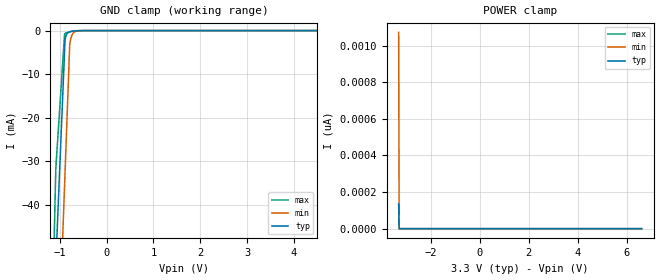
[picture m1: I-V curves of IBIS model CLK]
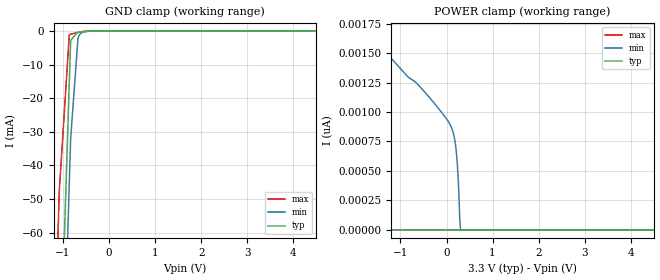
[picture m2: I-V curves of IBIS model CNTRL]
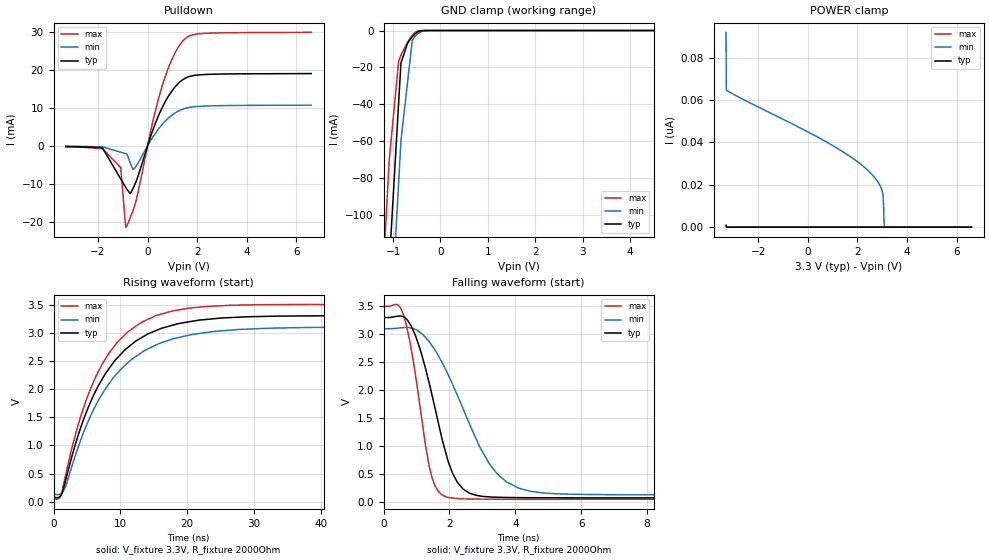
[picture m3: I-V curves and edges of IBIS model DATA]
|Texas Instruments Incorporated
| Marketing part#   Digital Voltage Range   Package-type   #pins
|   TPS544C20   3.1V -3.5V   LQFN   40
[IBIS Ver]   4.1
[File name]   tps544c20.ibs
[File Rev]   1.0
[Date]   02/18/2016
[Source]
| Texas Instruments Incorporated.
| 12500 TI Blvd
| Dallas, TX -75243
[Notes]   Revision History:
| Rev 1.0: 02/18/2016
| - Initial version of the model
| - Model generated from simulations in TISPICE
| - C_comp although listed in numerical order of value are
|   obtained from varying PVT conditions. For PVT conditions for
|   each specific value refer the buffer description under
|   respective [Model]. IBIS model user is responsible for using
|   appropriate C_comp to simulate for Signal Integrity.
| - Warnings regarding combined Non-monotonicity of various models have been
|   reviewd and considered minor and can be ignored.
[Disclaimer]
| This model is designed as an aid for customers of Texas Instruments.
| TI and its licensors and suppliers make no warranties, either expressed
| or implied, with respect to this  model, including the warranties of
| merchantability or fitness for a particular purpose. The model is
| provided solely on an "as is" basis. The entire risk as to its quality
| and performance is with the customer.
[Copyright]
 (C) Copyright 2016 Texas Instruments Incorporated.All rights reserved.
|   Device
[Component]   TPS544C20
[Manufacturer]   TI
[Package]
| variable   typ   min   max
R_pkg   0.2   0.16   0.24
L_pkg   1.5nH   1.2nH   1.8nH
C_pkg   0.4pF   0.32pF   0.48pF
[Pin]  signal_name   model_name   R_pin   L_pin   C_pin
1   CNTL   CNTRL   NA   NA   NA
2   ADDR1   NC   NA   NA   NA
3   ADDR0   NC   NA   NA   NA
4   DATA   DATA   NA   NA   NA
5   CLK   CLK   NA   NA   NA
6   SMBALERTB   SMBALERT   NA   NA   NA
7   BOOT   NC   NA   NA   NA
8   SW   NC   NA   NA   NA
9   SW   NC   NA   NA   NA
10   SW   NC   NA   NA   NA
11   SW   NC   NA   NA   NA
12   SW   NC   NA   NA   NA
13   AGNDSNS   GND   NA   NA   NA
14   GND   GND   NA   NA   NA
15   GND   GND   NA   NA   NA
16   GND   GND   NA   NA   NA
17   GND   GND   NA   NA   NA
18   GND   GND   NA   NA   NA
19   GND   GND   NA   NA   NA
20   GND   GND   NA   NA   NA
21   VIN   NC   NA   NA   NA
22   VIN   NC   NA   NA   NA
23   VIN   NC   NA   NA   NA
24   VIN   NC   NA   NA   NA
25   VIN   NC   NA   NA   NA
26   PGND   GND   NA   NA   NA
27   BP3   POWER   NA   NA   NA
28   BP6   POWER   NA   NA   NA
29   VDD   POWER   NA   NA   NA
30   BPEXT   NC   NA   NA   NA
31   VOUTS+   NC   NA   NA   NA
32   VOUTS-   NC   NA   NA   NA
33   DIFFO   NC   NA   NA   NA
34   FB   NC   NA   NA   NA
35   COMP   NC   NA   NA   NA
36   PGOOD   NC   NA   NA   NA
37   TSNS   NC   NA   NA   NA
38   AGND   GND   NA   NA   NA
39   MODE   NC   NA   NA   NA
40   RT   NC   NA   NA   NA
| Models and submodels in the file (4): CLK (Input), CNTRL (Input), DATA (I/O_open_drain), SMBALERT (Open_drain)
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|   Model
[Model]   CLK
Model_type   Input
Vinl = 0.99
Vinh = 2.31
|   typ   min   max
C_comp   0.057pF   0.055pF   0.060pF
[Voltage Range]   3.3   3.1   3.5
[Temperature Range]   25   125   -40
[Power Clamp Reference]   3.3   3.1   3.5
[GND Clamp Reference]   0   0   0
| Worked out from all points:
|   GND clamp passes 1 mA (typ) near -0.86 V on its own axis
[GND Clamp]
|   Voltage   I(typ)   I(min)   I(max)
-3.3V     -1.121A    -1.154A    -1.103A
-1.825V   -397.6mA   -433.8mA   -376.6mA
-1.082V   -53.42mA   -90.58mA   -31.68mA
-894.3mV  -4.553mA   -35.25mA   -727.9uA
-884.4mV  -1.981mA   -32.34mA   -661.1uA
-864.6mV  -1.187mA   -26.51mA   -557.5uA
-834.9mV  -611.3uA   -17.77mA   -438.9uA
-785.4mV  -279.6uA   -3.211mA   -286.8uA
-765.6mV  -218.9uA   -2.042mA   -236.7uA
-735.9mV  -154.8uA   -1.024mA   -172uA
-656.7mV  -57.61uA   -188.9uA   -58.46uA
6.6V      0A         0A         0A
[POWER Clamp]
|   Voltage   I(typ)   I(min)   I(max)
-3.3V     135.7pA    1.072nA    121.6pA
-3.28V    0A         0A         0A
-3.27V    0A         0A         0A
6.6V      0A         0A         0A
|   Model
[Model]   CNTRL
Model_type   Input
Vinl = 0.99
Vinh = 2.31
|   typ   min   max
C_comp   0.165pF   0.160pF   0.170pF
[Voltage Range]   3.3   3.1   3.5
[Temperature Range]   25   125   -40
[Power Clamp Reference]   3.3   3.1   3.5
[GND Clamp Reference]   0   0   0
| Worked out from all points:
|   GND clamp passes 1 mA (typ) near -0.73 V on its own axis
[GND Clamp]
|   Voltage   I(typ)   I(min)   I(max)
-3.3V     -1.153A    -1.202A    -1.125A
-1.825V   -428.1mA   -480.4mA   -397.5mA
-1.082V   -109.1mA   -144.2mA   -47.78mA
-864.6mV  -15.54mA   -45.57mA   -1.146mA
-844.8mV  -7.029mA   -36.61mA   -1.005mA
-834.9mV  -2.776mA   -32.12mA   -950.8uA
-696.3mV  -487uA     -5.994mA   -438.3uA
-676.5mV  -428.6uA   -2.262mA   -378.8uA
-636.9mV  -325.8uA   -1.005mA   -269.2uA
-577.5mV  -195.5uA   -390.3uA   -134.3uA
-260.7mV  -171.7nA   -2.829uA   -12.91nA
6.6V      0A         0A         0A
[POWER Clamp]
|   Voltage   I(typ)   I(min)   I(max)
-3.3V     157.7pA    6.207nA    121.7pA
-3.28V    0A         2.44nA     0A
-1.825V   0A         1.725nA    0A
-290.4mV  0A         1.086nA    0A
46.2mV    0A         914.4pA    0A
165mV     0A         791.8pA    0A
204.6mV   0A         690.8pA    0A
234.3mV   0A         559.5pA    0A
264mV     0A         343.2pA    0A
283.8mV   0A         126.7pA    0A
303.6mV   0A         0A         0A
6.6V      0A         0A         0A
|   Model
[Model]   DATA
Model_type   I/O_open_drain
Polarity   Non-Inverting
Enable   Active-Low
Vinl = 0.99
Vinh = 2.31
Vmeas = 1.65
Vref = 3.3
Cref = 1pF
Rref = 2000
|   typ   min   max
C_comp   1.711pF   1.609pF   1.803pF
[Voltage Range]   3.3   3.1   3.5
[Temperature Range]   25   125   -40
[Pullup Reference]   3.3   3.1   3.5
[Pulldown Reference]   0   0   0
[Power Clamp Reference]   3.3   3.1   3.5
[GND Clamp Reference]   0   0   0
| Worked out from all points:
|   slope of the pulldown table from 0 to 0.495 V, typ, clamps not added: 56.7 ohm
|   GND clamp passes 1 mA (typ) near -0.49 V on its own axis
|   falling waveform, V_fixture 3.3V, R_fixture 2000Ohm: 20-80 % time 818ps typ, 1.41ns min, 539ps max; typ from 3.3 V to 0.079 V
|   rising waveform, V_fixture 3.3V, R_fixture 2000Ohm: 20-80 % time 7.79ns typ, 8.48ns min, 7.08ns max; typ from 0.079 V to 3.3 V
[Pulldown]
|   Voltage   I(typ)   I(min)   I(max)
-3.3V     -205.5uA   -132.1uA   -271.9uA
-1.825V   -527uA     -305.2uA   -764.4uA
-1.082V   -8.73mA    -1.699mA   -5.761mA
-874.5mV  -11.03mA   -2.089mA   -21.39mA
-696.3mV  -12.6mA    -4.527mA   -18.87mA
-537.9mV  -10.51mA   -5.973mA   -16.1mA
165mV     3.269mA    1.839mA    5.096mA
570.9mV   9.793mA    5.493mA    15.34mA
986.7mV   14.45mA    8.065mA    22.78mA
1.422V    17.38mA    9.626mA    27.57mA
2.234V    18.7mA     10.41mA    29.51mA
6.6V      18.97mA    10.67mA    29.81mA
[GND Clamp]
|   Voltage   I(typ)   I(min)   I(max)
-3.3V     -1.18A     -1.238A    -1.146A
-1.825V   -455.3mA   -515.4mA   -419.6mA
-1.082V   -127mA     -173.7mA   -70.27mA
-884.4mV  -39.47mA   -82.63mA   -16.65mA
-834.9mV  -17.59mA   -59.85mA   -13.44mA
-696.3mV  -6.981mA   -28.24mA   -6.439mA
-597.3mV  -3.464mA   -5.667mA   -2.608mA
-557.7mV  -2.34mA    -3.882mA   -1.496mA
-498.3mV  -1.059mA   -2.198mA   -454.6uA
-369.6mV  -61.13uA   -384.9uA   -9.731uA
-191.4mV  -252.1nA   -8.629uA   0A
6.6V      0A         0A         0A
[POWER Clamp]
|   Voltage   I(typ)   I(min)   I(max)
-3.3V     925.8pA    91.96nA    369.2pA
-3.29V    462.9pA    64.65nA    184.6pA
590.7mV   0A         41.25nA    0A
1.541V    0A         34.62nA    0A
2.293V    0A         28.16nA    0A
2.709V    0A         23.19nA    0A
2.986V    0A         17.63nA    0A
3.036V    0A         14.33nA    0A
3.056V    0A         9.359nA    0A
3.066V    0A         4.25nA     0A
3.086V    0A         0A         0A
6.6V      0A         0A         0A
[Ramp]
R_load = 2000
|   typ   min   max
dV/dt_r   1.93263/7.79127e-09   1.78095/8.47977e-09   2.06772/7.08485e-09
dV/dt_f   1.93263/8.18406e-10   1.78095/1.40911e-09   2.06772/5.39276e-10
[Falling Waveform]
V_fixture = 3.3V
V_fixture_min = 3.1V
V_fixture_max = 3.5V
R_fixture = 2000Ohm
C_fixture = 0F
|   Time   V(typ)   V(min)   V(max)
0s        3.3V       3.1V       3.5V
532.3ps   3.325V     3.116V     3.451V
959.6ps   2.989V     3.088V     2.298V
1.465ns   1.926V     2.8V       448.7mV
1.667ns   1.405V     2.611V     189.8mV
2.173ns   432mV      2.002V     69.95mV
2.613ns   162.6mV    1.393V     59.96mV
3.448ns   90.67mV    510.4mV    55.56mV
5.617ns   80.54mV    146mV      53.92mV
100ns     78.94mV    131.6mV    53.76mV
[Rising Waveform]
V_fixture = 3.3V
V_fixture_min = 3.1V
V_fixture_max = 3.5V
R_fixture = 2000Ohm
C_fixture = 0F
|   Time   V(typ)   V(min)   V(max)
0s        78.94mV    131.6mV    53.76mV
1.025ns   102.2mV    141.5mV    89.3mV
1.606ns   287.9mV    215.4mV    363.1mV
3.346ns   1.05V      851.3mV    1.222V
4.853ns   1.572V     1.337V     1.795V
8.302ns   2.365V     2.097V     2.64V
12.37ns   2.859V     2.584V     3.122V
17.59ns   3.127V     2.881V     3.382V
32.18ns   3.292V     3.081V     3.499V
100ns     3.3V       3.1V       3.5V
